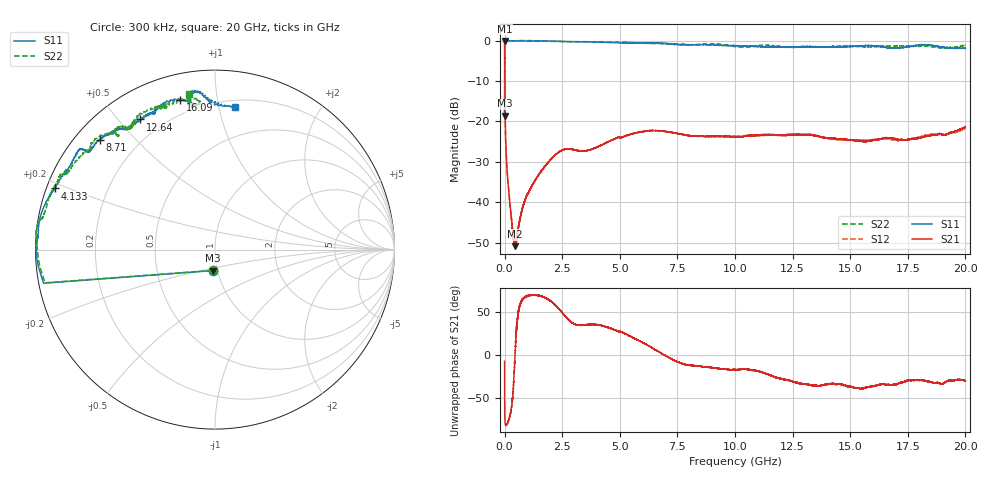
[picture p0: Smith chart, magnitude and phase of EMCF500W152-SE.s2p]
!EMCF500W152
!Johanson Technology Inc.
!www.johansontechnology.com
!Test Board Conditions:
!Substrate Type  RO4350B
!Substrate Thickness  6.6 mil
!Substrate Dk  3.66
!TL Type: GCPW
!TL Trace Width  13 mil
!TL Gap  7.5 mil
!PART MODE SINGLE ENDED (AKA BYPASS)
!DUT TOPOLOGY	SERIES-SHUNT
# MHz S  dB  R 50
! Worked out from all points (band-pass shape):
!   20001 points, 300 kHz to 20 GHz, reference 50 ohm
!   highest |S21| = -0.06 dB at 300 kHz (marker M1); lowest = -50.9 dB at 451.3 MHz (marker M2)
!   |S21| within 3 dB of the highest: start of sweep to 2.524 MHz
!   lowest |S11| = -18.6 dB at 300 kHz (marker M3), VSWR 1.27, Z = 47.5 - j11.3 ohm
!   |S11| at or under -10 dB: start of sweep to 1.035 MHz
!   |S22| runs from -18.7 to 0.0 dB; largest |S21 - S12| = 0.0039
!   S11 on the Smith chart (normalised r, x): 300 kHz: 0.95, -0.23; 4.133 GHz: 0.02, +0.18; 8.71 GHz: 0.07, +0.40; 12.64 GHz: 0.12, +0.57; 16.09 GHz: 0.13, +0.79; 20 GHz: 0.25, +1.12
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0.3  -18.59 -96.1  -0.06 -7.3  -0.05 -7.3  -18.70 -96.0
102.298  -0.04 -179.1  -31.60 -79.6  -31.58 -79.9  -0.10 -179.0
144.298  -0.04 -179.9  -34.89 -77.6  -34.81 -77.7  -0.09 -179.7
336.295  -0.03 179.0  -46.41 -52.8  -46.21 -52.0  -0.06 178.2
451.293  -0.04 178.3  -50.89 -2.6  -50.65 -1.0  -0.04 177.2
899.287  -0.08 176.1  -39.30 66.9  -39.33 67.6  0.01 174.0
1649.275  -0.07 171.9  -31.89 67.3  -31.84 67.5  -0.12 170.3
2474.263  -0.19 164.3  -27.23 49.8  -27.18 49.3  -0.24 168.4
3334.25  -0.28 161.7  -27.31 34.5  -27.35 34.5  -0.26 163.0
4133.238  -0.41 159.1  -26.08 34.6  -26.08 34.6  -0.37 158.3
6667.2  -0.60 143.0  -22.34 4.2  -22.30 4.0  -0.70 149.6
8710.169  -1.04 136.3  -23.71 -13.7  -23.77 -13.9  -0.84 140.1
10000.15  -1.30 129.8  -23.80 -16.9  -23.60 -16.6  -1.50 130.6
12637.11  -1.55 119.9  -23.31 -31.7  -23.18 -31.9  -1.59 123.9
13334.1  -1.55 115.1  -23.39 -35.0  -23.33 -35.5  -1.58 122.2
14424.08  -1.59 114.0  -24.39 -33.7  -24.45 -33.6  -1.42 121.5
15087.07  -1.45 112.5  -24.63 -37.3  -24.62 -36.0  -1.29 114.6
16091.06  -1.36 103.0  -24.62 -35.5  -24.49 -37.5  -1.47 109.1
16667.05  -1.79 99.0  -24.06 -34.2  -24.38 -35.0  -1.36 111.9
17367.04  -1.64 99.1  -24.63 -30.7  -24.65 -29.4  -1.40 110.5
18622.02  -1.28 94.7  -23.38 -32.0  -23.21 -33.2  -1.55 96.5
20000  -1.88 82.1  -21.37 -29.8  -21.71 -28.7  -1.16 99.4
